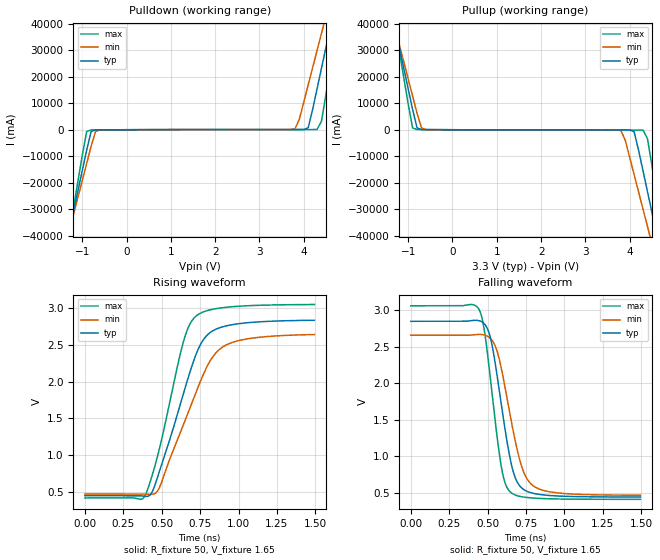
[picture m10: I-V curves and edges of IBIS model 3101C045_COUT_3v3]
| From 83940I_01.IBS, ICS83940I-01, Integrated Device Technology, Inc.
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[Model] 3101C045_COUT_3v3
Model_type   Output
Polarity   Non-Inverting
|   typ   min   max
C_comp   2pF   1.5pF   2.5pF
Vmeas = 1.65V
Rref = 50
Vref = 1.65V
|   typ   min   max
[Voltage range]   3.3V   3.135V   3.465V
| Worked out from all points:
|   slope of the pulldown table from 0 to 0.495 V, typ, clamps not added: 18.7 ohm
|   slope of the pullup table from 0 to 0.495 V, typ, clamps not added: 19.3 ohm
|   rising waveform, R_fixture 50, V_fixture 1.65: 20-80 % time 213ps typ, 250ps min, 171ps max; typ from 0.443 V to 2.84 V
|   falling waveform, R_fixture 50, V_fixture 1.65: 20-80 % time 109ps typ, 127ps min, 90.9ps max; typ from 2.84 V to 0.444 V
[pulldown]
|Voltage   I (typ)   I (min)   I (max)
-3.3V     -194.6A    -168.4A    -238.8A
-1.3V     -38.8A     -38.65A    -39.6A
-900mV    -7.64A     -12.71A    -689.3mA
-800mV    -712.3mA   -6.222A    -55.06mA
-600mV    -33.88mA   -54.97mA   -38.11mA
3.8V      62.42mA    258mA      72.56mA
4.1V      730.5mA    16.93A     72.88mA
4.3V      15.44A     29.9A      98.24mA
4.4V      23.23A     36.38A     3.253A
4.6V      38.8A      49.35A     23.17A
4.8V      54.38A     62.32A     43.08A
6.6V      194.6A     179.1A     222.4A
[pullup]
|Voltage   I (typ)   I (min)   I (max)
-3.3V     194.7A     168.4A     238.9A
-1.3V     38.81A     38.66A     39.61A
-900mV    7.643A     12.71A     695.5mA
-800mV    714.8mA    6.223A     61.06mA
-600mV    35.82mA    56.21mA    42.63mA
3.8V      -79.71mA   -273.3mA   -98.63mA
4.1V      -753.1mA   -16.95A    -101.1mA
4.3V      -15.47A    -29.92A    -132.1mA
4.4V      -23.26A    -36.41A    -3.291A
4.6V      -38.84A    -49.38A    -23.21A
4.8V      -54.42A    -62.35A    -43.13A
6.6V      -194.6A    -179.1A    -222.4A
[Ramp]
|   typ   min   max
dV/dt_r   1.925/0.31n   1.746/0.359n   2.127/0.254n
dV/dt_f   1.931/0.165n   1.757/0.197n   2.129/0.135n
[Rising Waveform]
R_fixture = 50
V_fixture = 1.65
V_fixture_max = 1.73
V_fixture_min = 1.57
C_fixture = 0.0p
| Time   typ   min   max
0s        443.3mV    467.1mV    412.4mV
388.1ps   434mV      466.7mV    432.1mV
433.1ps   477.8mV    461.1mV    687.3mV
482.5ps   760.1mV    543.1mV    1.061V
639.9ps   1.828V     1.405V     2.534V
678.8ps   2.099V     1.617V     2.767V
723.8ps   2.375V     1.861V     2.896V
824.2ps   2.684V     2.315V     2.985V
924.6ps   2.764V     2.506V     3.017V
1.494ns   2.839V     2.644V     3.054V
[Falling Waveform]
R_fixture = 50
V_fixture = 1.65
V_fixture_max = 1.73
V_fixture_min = 1.57
C_fixture = 0.0p
| Time   typ   min   max
0s        2.844V     2.654V     3.056V
445.1ps   2.852V     2.665V     3.002V
479.5ps   2.808V     2.657V     2.71V
523ps     2.576V     2.599V     1.968V
591.9ps   1.666V     2.173V     823.7mV
651.8ps   915.2mV    1.502V     505.5mV
684.8ps   681.2mV    1.159V     467.6mV
728.3ps   556.2mV    818.4mV    445.7mV
810.7ps   488.6mV    577.8mV    428mV
1.494ns   443.8mV    468.3mV    412.5mV
